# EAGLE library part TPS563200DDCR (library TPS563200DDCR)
17 V Input, 3A Synchronous Step-Down Regulator in SOT-23 with Advanced Eco-mode Source: Datasheet
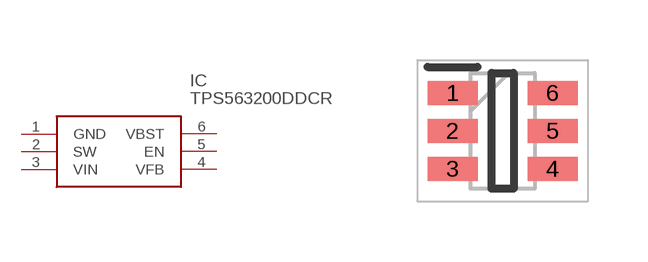
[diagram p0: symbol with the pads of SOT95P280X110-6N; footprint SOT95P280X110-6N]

Designator prefix IC

## TPS563200DDCR (Description: 17 V Input, 3A Synchronous Step-Down Regulator in SOT-23 with Advanced Eco-mode; Height: 1.1mm; Manufacturer_Name: Texas Instruments; Manufacturer_Part_Number: TPS563200DDCR; Mouser_Part_Number: 595-TPS563200DDCR; Mouser_Price-Stock: https://www.mouser.co.uk/ProductDetail/Texas-Instruments/TPS563200DDCR?qs=bT6MOr62zwLjxJIF4PA64g%3D%3D)  [SOT95P280X110-6N]
1  GND  pwr
2  SW
3  VIN  pwr
4  VFB  in
5  EN  in
6  VBST

## Footprint SOT95P280X110-6N (pad centres in mm)
TPS563200
smd 1.25 x 0.6: 1 -1.25,0.95; 2 -1.25,0; 3 -1.25,-0.95; 4 1.25,-0.95; 5 1.25,0; 6 1.25,0.95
